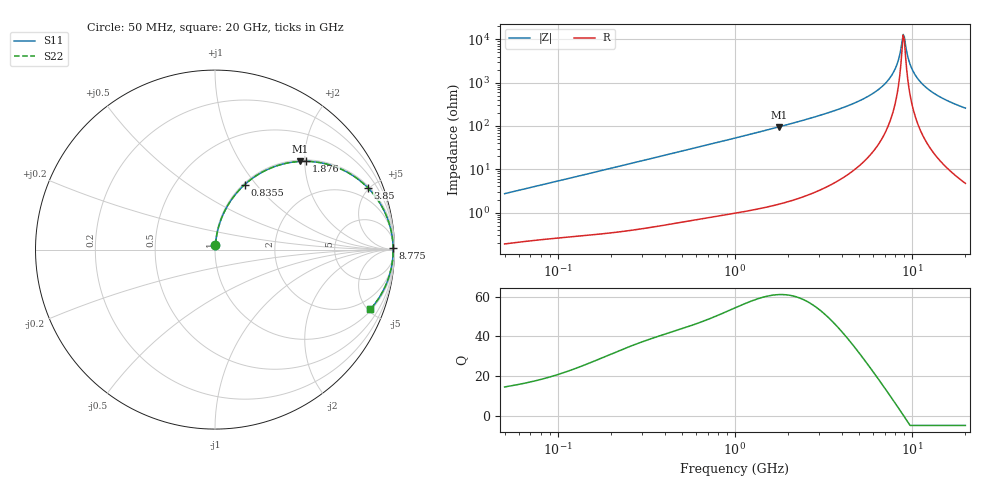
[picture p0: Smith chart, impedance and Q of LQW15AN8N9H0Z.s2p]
!Murata Part Number: LQW15AN8N9H0Z
!These Parameters are Measured in Series Mode Connection
!  o--[Z]--o
!Port1  Port2
!  o-------o
!Freq. Start=50[MHz] Stop=20[GHz], 401[Steps]
# Hz S RI R 50
!Freq.(Hz) S11(Real) S11(Imag) S21(Real) S21(Imag) S12(Real) S12(Imag) S22(Real) S22(Imag)
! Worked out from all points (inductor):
!   401 points, 50 MHz to 20 GHz, reference 50 ohm
!   read as one part in series: L = 8.6 nH near 51.52 MHz
!   highest Q = 61.2 at 1.767 GHz (marker M1), where L = 8.57 nH
!   self-resonance near 8.907 GHz
!   S11 on the Smith chart (normalised r, x): 50 MHz: 1.00, +0.05; 835.5 MHz: 1.02, +0.88; 1.876 GHz: 1.03, +2.03; 3.85 GHz: 1.11, +4.88; 8.775 GHz: open; 20 GHz: 1.09, -5.17
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5e7  0.00262 0.0271  0.9974 -0.0271  0.9974 -0.0271  0.00262 0.0271
1.364002e8  0.00806 0.0716  0.9919 -0.0716  0.9919 -0.0716  0.00806 0.0716
3.721004e8  0.0412 0.1866  0.9588 -0.1866  0.9588 -0.1866  0.0412 0.1866
8.354841e8  0.1659 0.3624  0.8341 -0.3624  0.8341 -0.3624  0.1659 0.3624
1e9  0.2207 0.4057  0.7793 -0.4057  0.7793 -0.4057  0.2207 0.4057
1.766834e9  0.4753 0.4913  0.5247 -0.4913  0.5247 -0.4913  0.4753 0.4913
1.875929e9  0.5072 0.4918  0.4928 -0.4918  0.4928 -0.4918  0.5072 0.4918
2.728004e9  0.7038 0.4478  0.2962 -0.4478  0.2962 -0.4478  0.7038 0.4478
3.850025e9  0.8506 0.3454  0.1494 -0.3454  0.1494 -0.3454  0.8506 0.3454
5.769027e9  0.9558 0.186  0.0442 -0.186  0.0442 -0.186  0.9558 0.186
6.701223e9  0.9768 0.123  0.0232 -0.123  0.0232 -0.123  0.9768 0.123
7.442007e9  0.9862 0.0786  0.0138 -0.0786  0.0138 -0.0786  0.9862 0.0786
8.141811e9  0.9909 0.0403  0.00909 -0.0403  0.00909 -0.0403  0.9909 0.0403
8.389408e9  0.9918 0.0275  0.00819 -0.0275  0.00819 -0.0275  0.9918 0.0275
8.774992e9  0.9925 0.00836  0.00745 -0.00836  0.00745 -0.00836  0.9925 0.00836
9.041845e9  0.9926 -0.00442  0.00738 0.00442  0.00738 0.00442  0.9926 -0.00442
9.600142e9  0.9918 -0.03  0.00822 0.03  0.00822 0.03  0.9918 -0.03
9.892087e9  0.9909 -0.0428  0.00913 0.0428  0.00913 0.0428  0.9909 -0.0428
1.050288e10  0.988 -0.0683  0.012 0.0683  0.012 0.0683  0.988 -0.0683
1.149051e10  0.9812 -0.1065  0.0188 0.1065  0.0188 0.1065  0.9812 -0.1065
1.438523e10  0.9503 -0.2013  0.0497 0.2013  0.0497 0.2013  0.9503 -0.2013
2e10  0.8652 -0.3324  0.1348 0.3324  0.1348 0.3324  0.8652 -0.3324
